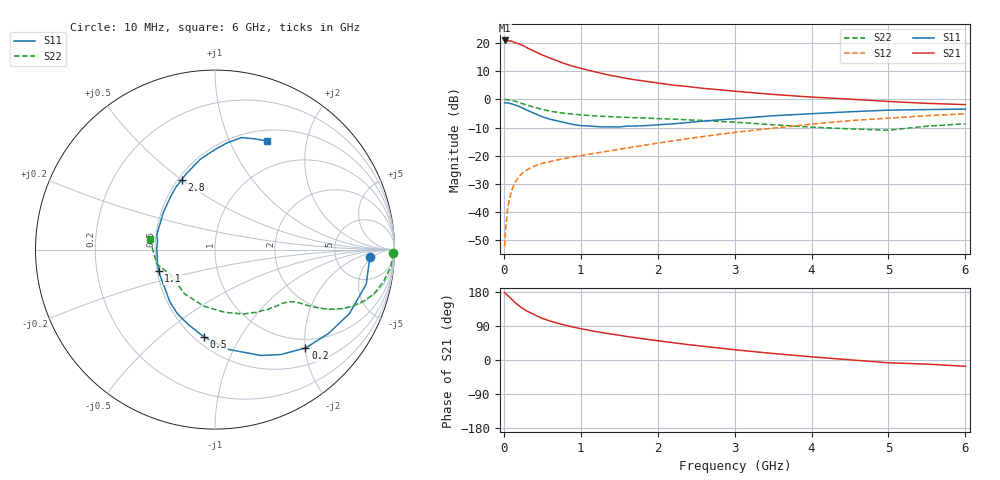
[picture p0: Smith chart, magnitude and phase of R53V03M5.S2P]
! SIEMENS Small Signal Semiconductors
! BFR183
! Si NPN RF Bipolar Junction Transistor in SOT23
! VCE = 3 V  IC = 3.5 mA
! Common Emitter S-Parameters:  May  1996
# GHz  S  MA  R  50
!  f  S11  S21  S12  S22
! GHz  MAG  ANG  MAG  ANG  MAG  ANG  MAG  ANG
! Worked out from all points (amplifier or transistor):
!   36 points, 10 MHz to 6 GHz, reference 50 ohm
!   highest |S21| = 20.8 dB at 10 MHz (marker M1)
!   |S21| within 3 dB of that: start of sweep to 333 MHz
!   unconditionally stable (mu >= 1): 1.183 GHz to 2.701 GHz
!   at 250 MHz: K = 0.33, MSG = 22.5 dB, |S12| = -26.0 dB
!   at 1.4 GHz: K = 1.06, MAG = 11.8 dB, |S12| = -18.2 dB
!   at 6 GHz: K = 0.89, MSG = 1.6 dB, |S12| = -5.1 dB
!   S11 on the Smith chart (normalised r, x): 10 MHz: 13, -4; 200 MHz: 0.81, -2.01; 500 MHz: 0.56, -0.71; 1.1 GHz: 0.51, -0.14; 2.8 GHz: 0.52, +0.50; 6 GHz: 0.63, +1.39
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0.01  0.8663 -2.7  11.01 178.2  0.0025 88.3  0.9934 -1.1
0.02  0.8615 -5.1  10.86 175.9  0.0045 88.3  0.9904 -2.3
0.05  0.8644 -12.8  10.87 170.1  0.0121 84.2  0.9843 -5.5
0.1  0.8297 -25.4  10.7 160.6  0.0242 77.4  0.9559 -10.7
0.15  0.7863 -36.5  10.02 150.9  0.0342 71.1  0.9208 -15.4
0.2  0.7449 -47.4  9.549 142.8  0.0434 66.4  0.8781 -19.0
0.25  0.6896 -58.0  8.918 135.3  0.0503 61.7  0.8296 -22.2
0.3  0.6428 -66.6  8.19 129.1  0.056 59.2  0.7879 -24.6
0.4  0.5605 -82.5  7.052 119.1  0.0662 54.7  0.7186 -27.6
0.5  0.4906 -97.1  6.089 109.9  0.0732 52.5  0.6605 -29.5
0.6  0.443 -109.7  5.368 102.9  0.079 51.2  0.6166 -30.7
0.7  0.4135 -120.5  4.753 97.0  0.0844 50.8  0.5865 -31.5
0.8  0.3847 -130.9  4.239 91.7  0.09 50.6  0.5626 -32.1
1.1  0.3365 -159.2  3.267 78.8  0.1059 52.4  0.5174 -34.2
1.3  0.3238 -174.0  2.814 71.6  0.1176 53.7  0.4974 -35.8
1.6  0.3339 166.1  2.335 62.0  0.1371 55.1  0.477 -39.2
2.2  0.3669 136.9  1.781 45.7  0.1834 55.8  0.4466 -48.3
2.8  0.4315 115.3  1.477 31.6  0.2394 53.2  0.4042 -60.6
3.5  0.5107 99.1  1.218 17.2  0.3079 47.0  0.3535 -81.2
4.5  0.6008 83.2  1.006 0.5  0.4186 35.2  0.2989 -124.8
5.5  0.657 69.7  0.846 -10.9  0.5118 22.1  0.3338 -166.2
6  0.6704 64.6  0.804 -16.6  0.5539 13.5  0.3678 171.0
